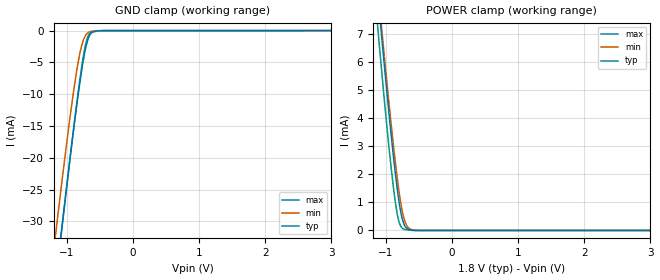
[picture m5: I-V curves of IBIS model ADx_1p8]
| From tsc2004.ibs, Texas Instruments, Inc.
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| Model 1.8 V ADx
[Model]   ADx_1p8
Model_type  Input
Vinl = 0.54
Vinh = 1.26
|   typ   min   max
|   (nom PVT)   (Fast PVT)   (slow PVT)
C_comp   6.66934E-12   6.16711E-12   6.88851E-12
| Where   nom PVT is  Nominal Process, 3.3V, 25C
|   Fast PVT is Strong Process, 3.6V, -40C
|   Slow PVT is Weak Process, 3.0V, 85C
|C_comp - from L-C Tank method, L = 1nH, peak frequency ~ 1.9G
|C_comp from frequency method, F = 10 MHz
[Model Spec]   | power 1.8, 1.65. 2 V
Vinl   0.54   0.495   0.6
Vinh   1.26   1.155   1.4
[Voltage Range]   1.8   1.65   2
[Temperature Range]   30   88   -40
|Ambient Temperature Range 27   85   -40
[Power Clamp Reference]   1.8   1.65   2
[GND Clamp Reference]   0   0   0
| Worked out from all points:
|   GND clamp passes 1 mA (typ) near -0.66 V on its own axis
|   POWER clamp passes 1 mA (typ) near -0.80 V on its own axis
[GND Clamp]
|   Voltage   I(typ)   I(min)   I(max)
-1.8V     -98.57mA   -90.01mA   -99.58mA
-1.173V   -39.87mA   -32.43mA   -40.22mA
-1.14V    -36.91mA   -29.54mA   -37.22mA
-1.084V   -31.8mA    -24.65mA   -32.05mA
-1.068V   -30.35mA   -23.25mA   -30.58mA
-947.6mV  -19.85mA   -13.38mA   -19.84mA
-834.3mV  -10.61mA   -5.378mA   -10.27mA
-741mV    -4.194mA   -1.301mA   -3.536mA
-678.8mV  -1.353mA   -336.9uA   -923.8uA
-622mV    -324.1uA   -113.1uA   -256.7uA
-461.7mV  -6.009uA   -7.918uA   -26.67uA
3.595V    0A         0A         0A
[POWER Clamp]
|   Voltage   I(typ)   I(min)   I(max)
-1.8V     26.66mA    26.45mA    26.02mA
-1.123V   8.404mA    8.654mA    7.217mA
-1.091V   7.575mA    7.848mA    6.36mA
-1.057V   6.716mA    7.016mA    5.495mA
-949.7mV  4.075mA    4.444mA    2.866mA
-876.7mV  2.426mA    2.822mA    1.345mA
-804.4mV  1.059mA    1.429mA    323.7uA
-748.8mV  372.2uA    639.9uA    73.92uA
-694.4mV  96.95uA    215uA      27.5uA
-660.8mV  39.34uA    98.7uA     18.71uA
-511.6mV  1.445uA    1.625uA    1.241uA
3.595V    0A         0A         0A
